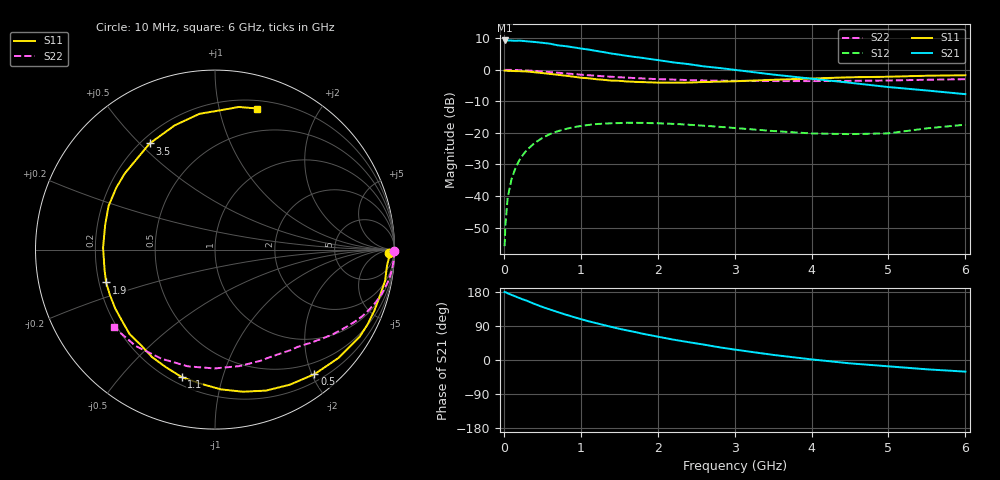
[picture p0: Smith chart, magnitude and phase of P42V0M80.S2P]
! SIEMENS Small Signal Semiconductors
! BFP182
! Si NPN RF Bipolar Junction Transistor in SOT143
! VCE = 2 V  IC = 0.8 mA
! Common Emitter S-Parameters:  March  1996
# GHz  S  MA  R  50
!  f  S11  S21  S12  S22
! GHz  MAG  ANG  MAG  ANG  MAG  ANG  MAG  ANG
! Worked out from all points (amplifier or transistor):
!   36 points, 10 MHz to 6 GHz, reference 50 ohm
!   highest |S21| = 9.3 dB at 10 MHz (marker M1)
!   |S21| within 3 dB of that: start of sweep to 1.127 GHz
!   unconditionally stable (mu >= 1): 2.741 GHz to end of sweep
!   at 250 MHz: K = 0.08, MSG = 18.0 dB, |S12| = -26.9 dB
!   at 1.4 GHz: K = 0.52, MSG = 11.0 dB, |S12| = -17.0 dB
!   at 6 GHz: K = 1.13, MAG = 2.6 dB, |S12| = -17.4 dB
!   S11 on the Smith chart (normalised r, x): 10 MHz: 51, -32; 500 MHz: 0.31, -2.04; 1.1 GHz: 0.24, -0.74; 1.9 GHz: 0.23, -0.14; 3.5 GHz: 0.23, +0.54; 6 GHz: 0.27, +1.31
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0.01  0.9722 -1.0  2.92 179.6  0.0016 83.0  0.9974 -0.3
0.02  0.9721 -2.1  2.912 179.1  0.0034 88.6  0.9968 -0.8
0.05  0.9626 -5.3  2.919 176.0  0.0094 87.6  0.9976 -1.9
0.1  0.9634 -10.4  2.906 171.9  0.0185 81.7  0.9964 -3.9
0.15  0.9538 -15.8  2.879 167.8  0.0274 80.2  0.9932 -5.8
0.2  0.9506 -21.0  2.903 163.6  0.0366 76.6  0.9885 -7.8
0.25  0.9467 -26.3  2.87 159.7  0.0451 73.9  0.9826 -9.8
0.4  0.9148 -41.4  2.763 147.8  0.0691 64.1  0.9603 -15.0
0.5  0.888 -51.4  2.681 140.1  0.0831 58.0  0.941 -18.4
0.6  0.8605 -61.0  2.595 133.2  0.0958 52.1  0.9199 -21.6
0.8  0.8069 -78.9  2.374 120.0  0.1149 42.0  0.8784 -27.0
1.1  0.7339 -104.7  2.096 102.3  0.1337 29.1  0.8204 -34.0
1.3  0.6937 -120.5  1.906 92.2  0.1405 21.7  0.7891 -38.0
1.5  0.6694 -135.3  1.74 82.4  0.1431 15.6  0.7618 -41.5
1.9  0.6337 -163.2  1.484 65.6  0.1431 5.7  0.7202 -48.2
2.2  0.6236 179.0  1.312 53.9  0.1392 0.0  0.7006 -53.1
2.8  0.6492 147.9  1.069 33.6  0.125 -7.3  0.6718 -63.8
3.5  0.6944 121.6  0.841 13.5  0.1071 -9.4  0.6632 -78.3
4.5  0.7616 96.5  0.623 -8.9  0.0956 1.2  0.6677 -103.0
5  0.7768 87.8  0.533 -16.7  0.0984 11.2  0.6771 -116.0
5.5  0.8057 80.5  0.47 -24.6  0.1181 14.3  0.6957 -129.5
6  0.8203 73.4  0.411 -30.7  0.1349 13.9  0.71 -142.4
